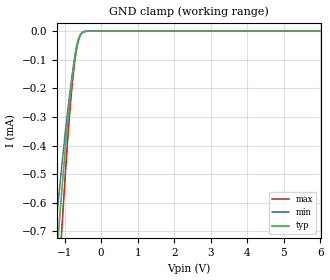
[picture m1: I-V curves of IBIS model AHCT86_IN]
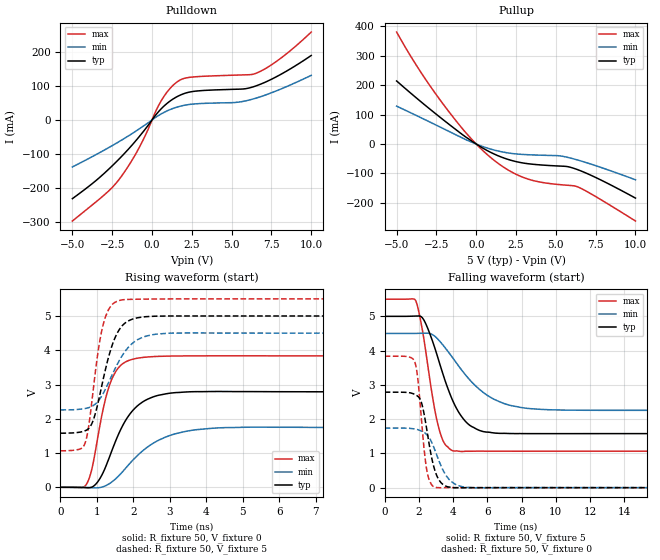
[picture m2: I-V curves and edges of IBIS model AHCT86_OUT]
| TEXAS INSTRUMENTS INCORPORATED
| Standard Linear and Logic Group
| IBIS Model of SN74AHCT86
| QUADRUPLE 2-INPUT EXCLUSIVE-OR GATES
| This file contains package information for the following:
|  SOIC 14-pin (D) package as [Component] AHCT86_D
|  SSOP 14-pin (DB) package as [Component] AHCT86_DB
|  TVSOP 14-pin (DGV) package as [Component] AHCT86_DGV
|  PDIP 14-pin (N) package as [Component] AHCT86_N
|  TSSOP 14-pin (PW) package as [Component] AHCT86_PW
| This device can be powered at the following Vccs:
|  5.0 volt Vcc
| This file provides unique models under the [Model Selector] for each Vcc.
| For operation at a specific Vcc, select the appropriate model after each
| [Model Selector] keyword.
[IBIS Ver]   3.2
[Comment char]  |_char
[File Name]   ahct86.ibs
[File Rev]   1.1 | c_die
[Date]   October 19, 2000
[Source]   Data created from TI-SPICE simulations at TI-SLL.
[Notes]   The following is an IBIS list for the AHCT86.
   Please contact sllibis@ti.com with questions and
   comments concerning SLL IBIS models.
   -To comply with the data sheet we omitted the Vref
   and Rref from the Output Model
   -As there is no power clamp diode in the Input Model,
   we removed the Pwr Clamp table data from the Input Models
[Disclaimer] Property of Texas Instruments Incorporated.  Unauthorized
   reproduction and/or distribution is strictly prohibited.
   This product is protected under copyright law.
   Created  2000, (C) Copyright  2000, Texas Instruments Inc.,
   All Rights Reserved
   UNLESS THERE IS A SIGNED, WRITTEN AGREEMENT TO THE
   CONTRARY, TEXAS INSTRUMENTS (TI) IS PROVIDING THE IBIS
   MODELS  AND WITHOUT ANY WARRANTY, EXPRESSED OR
   IMPLIED.  TI assumes no liability for:
   1) the accuracy of the IBIS models provided to your
   company;
   2) the proper functioning of these IBIS Models in your
   design or for any resulting applications; or
   3) infringement of patents, copyrights or intellectual
   property rights resulting from your use of these IBIS
   models.
   TI provides IBIS Models as a service to our customers.
   You and your company shall not distribute, sell or give
   these models to anyone else without prior written
   permission from TI.
   TI reserves the right to make changes to our products or
   to discontinue any semiconductor product or service
   without notice, and advises our customers to obtain the
   latest version of relevant information to verify, before
   placing orders, that the information being relied on is
   current.
   Please be aware that your receipt and use of the IBIS
   information provided shall serve as acceptance of these
   terms and conditions.  If you do not accept these terms,
   you should return or destroy the IBIS models and any
   other accompanying information immediately.
| Component AHCT86_D 14-pin SOIC
[Component]   AHCT86_D
[Manufacturer]   Texas Instruments, Inc.
[Package]
|   typ   min   max
R_pkg   3.100e-02   2.800e-02   3.400e-02
L_pkg   3.109e-09   2.462e-09   3.889e-09
C_pkg   4.730e-13   3.630e-13   6.280e-13
[Pin]   signal_name   model_name   R_pin   L_pin   C_pin
1   1A   AHCT86_IN   3.300e-02   3.854e-09   6.220e-13
2   1B   AHCT86_IN   3.200e-02   3.188e-09   4.730e-13
3   1Y   AHCT86_OUT   2.800e-02   2.462e-09   3.770e-13
4   2A   AHCT86_IN   3.100e-02   2.596e-09   3.630e-13
5   2B   AHCT86_IN   2.800e-02   2.521e-09   3.720e-13
6   2Y   AHCT86_OUT   3.400e-02   3.250e-09   4.760e-13
7   GND   GND   3.400e-02   3.889e-09   6.280e-13
8   3Y   AHCT86_OUT   3.400e-02   3.889e-09   6.280e-13
9   3A   AHCT86_IN   3.400e-02   3.250e-09   4.760e-13
10   3B   AHCT86_IN   2.800e-02   2.521e-09   3.720e-13
11   4Y   AHCT86_OUT   3.100e-02   2.596e-09   3.640e-13
12   4A   AHCT86_IN   2.800e-02   2.462e-09   3.770e-13
13   4B   AHCT86_IN   3.200e-02   3.188e-09   4.730e-13
14   VCC   POWER   3.300e-02   3.854e-09   6.220e-13
| Component AHCT86_DB 14-pin SSOP
[Component]   AHCT86_DB
[Manufacturer]   Texas Instruments, Inc.
[Package]
|   typ   min   max
R_pkg   4.400e-02   4.100e-02   4.600e-02
L_pkg   3.551e-09   3.258e-09   3.927e-09
C_pkg   4.020e-13   3.600e-13   4.210e-13
[Pin]   signal_name   model_name   R_pin   L_pin   C_pin
1   1A   AHCT86_IN   4.600e-02   3.927e-09   4.080e-13
2   1B   AHCT86_IN   4.400e-02   3.587e-09   4.210e-13
3   1Y   AHCT86_OUT   4.100e-02   3.289e-09   3.980e-13
4   2A   AHCT86_IN   4.200e-02   3.258e-09   3.600e-13
5   2B   AHCT86_IN   4.100e-02   3.286e-09   4.030e-13
6   2Y   AHCT86_OUT   4.400e-02   3.586e-09   4.210e-13
7   GND   GND   4.600e-02   3.927e-09   4.080e-13
8   3Y   AHCT86_OUT   4.600e-02   3.927e-09   4.080e-13
9   3A   AHCT86_IN   4.400e-02   3.586e-09   4.210e-13
10   3B   AHCT86_IN   4.100e-02   3.286e-09   4.030e-13
11   4Y   AHCT86_OUT   4.300e-02   3.258e-09   3.600e-13
12   4A   AHCT86_IN   4.100e-02   3.289e-09   3.980e-13
13   4B   AHCT86_IN   4.400e-02   3.587e-09   4.210e-13
14   VCC   POWER   4.600e-02   3.927e-09   4.080e-13
| Component AHCT86_DGV 14-pin TVSOP
[Component]   AHCT86_DGV
[Manufacturer]   Texas Instruments, Inc.
[Package]
|   typ   min   max
R_pkg   3.500e-02   2.000e-02   4.500e-02
L_pkg   2.499e-09   2.077e-09   2.966e-09
C_pkg   3.610e-13   3.050e-13   4.160e-13
[Pin]   signal_name   model_name   R_pin   L_pin   C_pin
1   1A   AHCT86_IN   2.700e-02   2.717e-09   3.730e-13
2   1B   AHCT86_IN   3.700e-02   2.434e-09   3.980e-13
3   1Y   AHCT86_OUT   3.400e-02   2.200e-09   3.160e-13
4   2A   AHCT86_IN   2.000e-02   2.077e-09   3.090e-13
5   2B   AHCT86_IN   3.000e-02   2.147e-09   3.050e-13
6   2Y   AHCT86_OUT   4.200e-02   2.580e-09   4.080e-13
7   GND   GND   3.900e-02   2.921e-09   3.850e-13
8   3Y   AHCT86_OUT   3.300e-02   2.841e-09   3.800e-13
9   3A   AHCT86_IN   4.200e-02   2.611e-09   4.100e-13
10   3B   AHCT86_IN   3.800e-02   2.331e-09   3.290e-13
11   4Y   AHCT86_OUT   2.600e-02   2.223e-09   3.190e-13
12   4A   AHCT86_IN   3.400e-02   2.259e-09   3.130e-13
13   4B   AHCT86_IN   4.500e-02   2.681e-09   4.160e-13
14   VCC   POWER   4.200e-02   2.966e-09   3.860e-13
| Component AHCT86_N 14-pin PDIP
[Component]   AHCT86_N
[Manufacturer]   Texas Instruments, Inc.
[Package]
|   typ   min   max
R_pkg   4.500e-02   3.700e-02   6.300e-02
L_pkg   5.407e-09   3.922e-09   6.942e-09
C_pkg   3.890e-13   2.050e-13   6.040e-13
[Pin]   signal_name   model_name   R_pin   L_pin   C_pin
1   1A   AHCT86_IN   6.300e-02   6.942e-09   6.040e-13
2   1B   AHCT86_IN   3.700e-02   6.200e-09   4.060e-13
3   1Y   AHCT86_OUT   4.200e-02   4.389e-09   3.220e-13
4   2A   AHCT86_IN   3.800e-02   3.922e-09   2.050e-13
5   2B   AHCT86_IN   3.900e-02   4.301e-09   2.980e-13
6   2Y   AHCT86_OUT   3.800e-02   5.329e-09   3.560e-13
7   GND   GND   5.300e-02   6.510e-09   5.440e-13
8   3Y   AHCT86_OUT   5.300e-02   6.437e-09   5.390e-13
9   3A   AHCT86_IN   3.900e-02   5.352e-09   3.470e-13
10   3B   AHCT86_IN   4.200e-02   4.473e-09   2.970e-13
11   4Y   AHCT86_OUT   4.400e-02   4.326e-09   2.250e-13
12   4A   AHCT86_IN   4.200e-02   4.295e-09   2.800e-13
13   4B   AHCT86_IN   4.200e-02   6.318e-09   4.180e-13
14   VCC   POWER   6.100e-02   6.900e-09   6.030e-13
| Component AHCT86_PW 14-pin TSSOP
[Component]   AHCT86_PW
[Manufacturer]   Texas Instruments, Inc.
[Package]
|   typ   min   max
R_pkg   3.200e-02   2.900e-02   3.500e-02
L_pkg   2.378e-09   2.170e-09   2.680e-09
C_pkg   3.140e-13   2.700e-13   3.350e-13
[Pin]   signal_name   model_name   R_pin   L_pin   C_pin
1   1A   AHCT86_IN   3.300e-02   2.618e-09   3.300e-13
2   1B   AHCT86_IN   3.100e-02   2.313e-09   3.170e-13
3   1Y   AHCT86_OUT   3.000e-02   2.310e-09   3.140e-13
4   2A   AHCT86_IN   3.100e-02   2.173e-09   2.720e-13
5   2B   AHCT86_IN   3.000e-02   2.204e-09   3.090e-13
6   2Y   AHCT86_OUT   3.200e-02   2.315e-09   3.170e-13
7   GND   GND   3.500e-02   2.680e-09   3.350e-13
8   3Y   AHCT86_OUT   3.300e-02   2.640e-09   3.330e-13
9   3A   AHCT86_IN   3.400e-02   2.347e-09   3.190e-13
10   3B   AHCT86_IN   2.900e-02   2.277e-09   3.130e-13
11   4Y   AHCT86_OUT   3.100e-02   2.170e-09   2.700e-13
12   4A   AHCT86_IN   3.100e-02   2.244e-09   3.110e-13
13   4B   AHCT86_IN   3.300e-02   2.343e-09   3.210e-13
14   VCC   POWER   3.500e-02   2.657e-09   3.320e-13
| Models and submodels in the file (2): AHCT86_IN (Input), AHCT86_OUT (Output)
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| Model AHCT86_IN
[Model]   AHCT86_IN
Model_type  Input
Vinl =   0.8
Vinh =   2.0
| variable   typ   min   max
C_comp   0.84pF   0.77pF   0.91pF
[Temperature Range]   40   100   -40
| Ambient temperature   25   85   -40
[Voltage range]   5   4.5   5.5
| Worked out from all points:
|   GND clamp passes 1 mA (typ) near -1.34 V on its own axis
[GND Clamp]
| AHCT86_IN
|   Voltage   I(typ)   I(min)   I(max)
-5V       -8.966mA   -7.191mA   -10.36mA
-1.27V    -883uA     -731.2uA   -1.114mA
-1.215V   -789.1uA   -655.8uA   -993.6uA
-1.16V    -697.2uA   -581.9uA   -875uA
-1.105V   -607.6uA   -509.8uA   -758.5uA
-1.065V   -543.9uA   -458.6uA   -675.4uA
-880mV    -271.8uA   -241.5uA   -322.3uA
-805mV    -177.1uA   -166.7uA   -208.2uA
-740mV    -107.3uA   -110.6uA   -127.9uA
-620mV    -27.63uA   -34.06uA   -32.68uA
-485mV    -3.248uA   -2.795uA   -2.776uA
6.005V    7.954nA    367.8pA    85.01nA
[Model]   AHCT86_OUT
Model_type  Output
|Vref =   0.0
|Rref =   1000
Cref =   50p
Vmeas =   1.5
| variable   typ   min   max
C_comp   12.69pF   11.14pF   14.47pF
| C_pullup   12.55pF   11.41pF   13.70pF
| C_pulldown   12.83pF   11.14pF   14.47pF
[Temperature Range]   40   100   -40
| Ambient temperature   25   85   -40
[Voltage range]   5   4.5   5.5
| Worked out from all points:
|   slope of the pulldown table from 0 to 0.75 V, typ, clamps not added: 18.4 ohm
|   slope of the pullup table from 0 to 0.75 V, typ, clamps not added: 31.3 ohm
|   rising waveform, R_fixture 50, V_fixture 0: 20-80 % time 749ps typ, 1.12ns min, 468ps max; typ from 0 V to 2.79 V
|   falling waveform, R_fixture 50, V_fixture 5: 20-80 % time 1.49ns typ, 2.38ns min, 862ps max; typ from 5 V to 1.58 V
|   rising waveform, R_fixture 50, V_fixture 5: 20-80 % time 493ps typ, 679ps min, 344ps max; typ from 1.58 V to 5 V
|   falling waveform, R_fixture 50, V_fixture 0: 20-80 % time 629ps typ, 921ps min, 427ps max; typ from 2.79 V to 0 V
[Pulldown]
| AHCT86_OUT
|   Voltage   I(typ)   I(min)   I(max)
-5V       -230.8mA   -137.8mA   -296.4mA
-2.86V    -150.5mA   -84.8mA    -214.2mA
-2.005V   -111.5mA   -61.75mA   -170.5mA
-800mV    -48.67mA   -25.99mA   -80.61mA
570mV     32.43mA    17.56mA    55.68mA
1.025V    51.64mA    28.26mA    86.54mA
1.515V    66.87mA    36.88mA    109.5mA
2.415V    82.42mA    45.88mA    125.3mA
5.245V    90.09mA    51.47mA    131.6mA
6.51V     99.62mA    63.76mA    136.6mA
8.02V     132mA      89.39mA    178.8mA
10V       189.2mA    130.9mA    258mA
[Pullup]
| AHCT86_OUT
|   Voltage   I(typ)   I(min)   I(max)
-5V       214.5mA    128.9mA    380.9mA
-3.525V   146.1mA    90.86mA    248mA
-1.875V   74.06mA    47.29mA    121.1mA
-335mV    12.04mA    7.527mA    19.25mA
1.105V    -33.46mA   -20.16mA   -54.63mA
2.17V     -55.08mA   -31.59mA   -93.51mA
3.235V    -66.79mA   -36.28mA   -118.9mA
5.17V     -74.69mA   -39.77mA   -137.6mA
6.055V    -81.31mA   -49.61mA   -141.5mA
6.395V    -87.69mA   -54.73mA   -146.2mA
7.025V    -101.8mA   -65.14mA   -163.7mA
10V       -183.8mA   -121.6mA   -261.7mA
[Ramp]
| AHCT86_OUT
| variable   typ   min   max
dV/dt_r   1.69/7.63E-10   1.06/1.15E-09   2.31/4.76E-10
dV/dt_f   2.06/1.53E-09   1.35/2.46E-09   2.67/8.84E-10
R_load = 50
[Rising Waveform]
| AHCT86_OUT
R_fixture =   50
C_fixture =   0
L_fixture =   0
V_fixture =   0
V_fixture_min = 0
V_fixture_max = 0
|   Time   V(typ)   V(min)   V(max)
0s        -230.6uV   -215.5uV   -195.4uV
710ps     -12.58mV   -5.003mV   85.84mV
860ps     5.488mV    -11.06mV   530.9mV
1.05ns    202.7mV    -11.34mV   1.619V
1.44ns    1.155V     182.4mV    3.232V
1.87ns    2.091V     659.5mV    3.701V
2.385ns   2.57V      1.174V     3.804V
3.465ns   2.784V     1.639V     3.835V
5.2ns     2.793V     1.755V     3.837V
50ns      2.787V     1.74V      3.836V
[Falling Waveform]
| AHCT86_OUT
R_fixture =   50
C_fixture =   0
L_fixture =   0
V_fixture =   5
V_fixture_min = 4.5
V_fixture_max = 5.5
|   Time   V(typ)   V(min)   V(max)
0s        5V         4.5V       5.5V
1.82ns    5.008V     4.503V     5.447V
2.325ns   4.86V      4.507V     4.226V
3.135ns   3.747V     4.319V     1.791V
3.5ns     3.167V     4.103V     1.285V
4.035ns   2.474V     3.747V     1.07V
4.745ns   1.92V      3.277V     1.063V
5.585ns   1.661V     2.848V     1.065V
9.11ns    1.576V     2.285V     1.063V
50ns      1.579V     2.258V     1.065V
[Rising Waveform]
| AHCT86_OUT
R_fixture =   50
C_fixture =   0
L_fixture =   0
V_fixture =   5
V_fixture_min = 4.5
V_fixture_max = 5.5
|   Time   V(typ)   V(min)   V(max)
0s        1.579V     2.258V     1.065V
665ps     1.646V     2.298V     1.264V
765ps     1.708V     2.322V     1.723V
905ps     1.978V     2.389V     2.904V
1.185ns   3.219V     2.766V     4.805V
1.45ns    4.245V     3.357V     5.366V
1.73ns    4.757V     3.904V     5.476V
2.25ns    4.97V      4.377V     5.493V
3.13ns    5.001V     4.503V     5.499V
50ns      5V         4.5V       5.5V
[Falling Waveform]
| AHCT86_OUT
R_fixture =   50
C_fixture =   0
L_fixture =   0
V_fixture =   0
V_fixture_min = 0
V_fixture_max = 0
|   Time   V(typ)   V(min)   V(max)
0s        2.787V     1.74V      3.836V
1.75ns    2.723V     1.712V     3.682V
1.92ns    2.672V     1.694V     3.235V
2.135ns   2.499V     1.654V     2.07V
2.455ns   1.708V     1.549V     527.7mV
2.65ns    1.122V     1.416V     162.9mV
3.03ns    365.6mV    968.5mV    1.831mV
3.845ns   10.41mV    198.1mV    1.567mV
5.165ns   -511.9uV   -4.312mV   -148.9uV
50ns      -230.5uV   -215.4uV   -195.3uV
